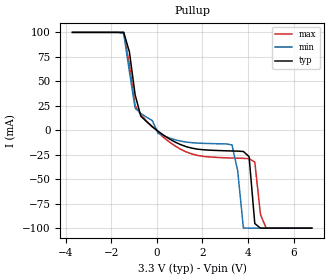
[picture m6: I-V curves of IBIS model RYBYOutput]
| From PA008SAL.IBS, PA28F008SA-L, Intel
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|****************Ready/Busy Output Model*****************************
[Model]   RYBYOutput
Model_type   Output
|   For RY/BY# pin 36
Vinl = 0.8V
Vinh = 2.0V
| Variable   typ   min   max
C_comp   9.61p   NA   11.6p
[Voltage Range]   3.3V   3.0V   3.6V
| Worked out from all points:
|   slope of the pullup table from 0 to 0.495 V, typ, clamps not added: 62 ohm
[Pulldown]
| [Pullup] and [Pulldown] IV curves include only the current through
| the channels of output driver transistors when outputs are enabled
| with OE# = VIL.  Although the output driver transistors have np and
| pn diodes inherently created by CMOS IC fabrication between the
| drain and bulk of n-channel and p-channel CMOS transistors,
| the current through these junction diodes is not included in
| [Pullup] or [Pulldown].  Instead that drain/bulk diode current is
| included in the [POWER_clamp] or [GND_clamp] sections, which are
| not dependent on the state of OE# or output data value.  The RY/BY#
| Pulldown information is not provided for this device.  The table
| below is for the compatibility with some IBIS parsers.
|Voltage  I(typ)   I(min)   I(max)
-3.3V     0A         0A         0A
0V        0A         0A         0A
3.3V      0A         0A         0A
6.6V      0A         0A         0A
[GND_clamp]
| The RY/BY# pin is always active and does NOT float to tri-state when
| the chip is deselected or when the data outputs are disabled.
| Therefore, the table below is included for the compatibility with
| some IBIS parsers.
|Voltage  I(typ)   I(min)   I(max)
-3.3V     0A         0A         0A
0V        0A         0A         0A
3.3V      0A         0A         0A
6.6V      0A         0A         0A
[Pullup]
| (Voltages for [Pullup] and [POWER_clamp] are specified with
| negative respect to Vcc.  Reference the IBIS documentation
| for more information regarding Vtable = Vcc - Voutput.
| This method keeps -Vds constant for the values in all three
| columns across a line of the table.)
| [Pullup] and [Pulldown] IV curves include only the current through
| the channels of output driver transistors when outputs are enabled
| with OE# = VIL.  Although the output driver transistors have np and
| pn diodes inherently created by CMOS IC fabrication between the
| drain and bulk of n-channel and p-channel CMOS transistors,
| the current through these junction diodes is not included in
| [Pullup] or [Pulldown].  Instead that drain/bulk diode current is
| included in the [POWER_clamp] or [GND_clamp] sections, which are
| not dependent on the state of OE# or output data value.
|Voltage  I(typ)   I(min)   I(max)
-3.7V     100mA      100mA      100mA
-1.45V    100mA      98.79mA    100mA
-950mV    36.25mA    22.64mA    25.21mA
50mV      -865uA     -3.011mA   -2.153mA
3.3V      -21.16mA   -14.95mA   -28.38mA
3.55V     -21.31mA   -41.39mA   -28.57mA
3.8V      -21.68mA   -99.84mA   -28.73mA
4.05V     -26.99mA   -100mA     -28.98mA
4.3V      -95.32mA   -100mA     -32.49mA
4.55V     -100mA     -100mA     -86.15mA
4.8V      -100mA     -100mA     -100mA
6.8V      -100mA     -100mA     -100mA
[POWER_clamp]
| The RY/BY# pin is always active and does NOT float to tri-state when
| the chip is deselected or when the data outputs are disabled.
| Therefore, the table below is included for the compatibility with
| some IBIS parsers.
|Voltage  I(typ)   I(min)   I(max)
-3.3V     0A         0A         0A
0V        0A         0A         0A
3.3V      0A         0A         0A
6.6V      0A         0A         0A
[Ramp]
| The RY/BY# Ramp information is not provided for this device.  The table
| below is for the compatibility with some IBIS parsers.
| Variable   typ   min   max
 dV/dt_r   0V/0ns   0V/0ns   0V/0ns
 dV/dt_f   0V/0ns   0V/0ns   0V/0ns
